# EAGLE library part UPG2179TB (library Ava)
The μPG2179TB is a GaAs MMIC L, S-band SPDT (Single Pole Double Throw) switch for mobile phone and other L, S-band applications. This device operates with dual control voltages of 2.5 to 5.3 V. This device can operate from 0.05 to 3.0 GHz, with low insertion loss and high isolation. http://datasheet.octopart.com/UPG2179TB-E4-A-NEC-datasheet-26379.pdf Layout by Anthony Stirk M0UPU UNTESTED
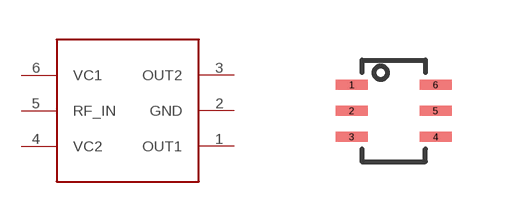
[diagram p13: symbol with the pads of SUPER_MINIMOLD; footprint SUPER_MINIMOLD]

Designator prefix -

## UPG2179TB  [SUPER_MINIMOLD]
1  OUT1
2  GND
3  OUT2
4  VC2
5  RF_IN
6  VC1

## Footprint SUPER_MINIMOLD (pad centres in mm)
smd 0.8 x 0.25: 1 -1.05,0.65; 2 -1.05,0; 3 -1.05,-0.65; 4 1.05,-0.65; 5 1.05,0; 6 1.05,0.65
